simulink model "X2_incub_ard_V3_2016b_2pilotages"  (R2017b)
settings: Solver=ode45  StartTime=0.0  StopTime=35*3600  RelTol=1e-3  EnableMultiTasking=on
undefined symbols (not defined in the file or in its folder): a12fe90b, a1c04bd6127d, a1fc367dfb9e, a2a0ec7e, a4c8, a889, a952, adec, aeaa, af92, b19e, b27f, b35c, b3e0, b3e1, beff, c20252f1455d, c375904d, c5628deb, c6119d757cc9, circulargauge, continuousknob, d0c8, d78370d7, e8b45f5d51c6, eec73065, f50e, f641dc3b1927, fb31cb14, fbd800df, fec15dcb, ff27feb4, lamp, lineargauge, ninetydegreegauge, rockerswitch, semicirculargauge, serial, X2_incub_ard_V3_2016b_2pilotages
libraries: instrumentlib x4, powerlib_meascontrol x1, simulink x1, visionstatistics x1

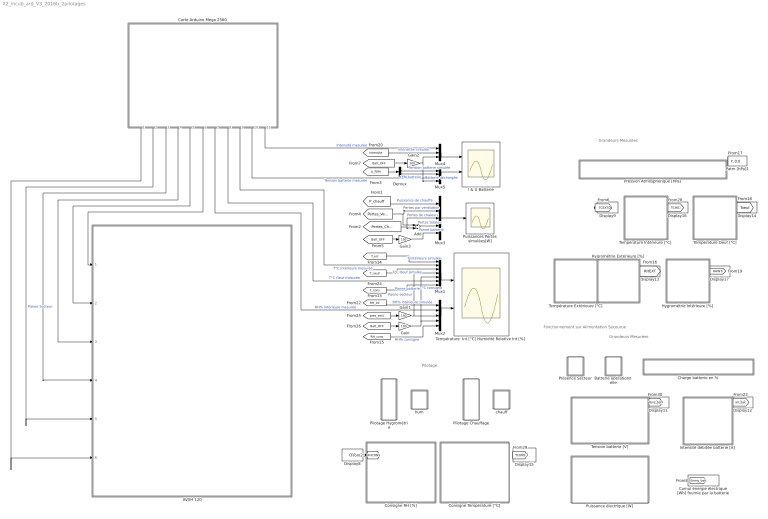
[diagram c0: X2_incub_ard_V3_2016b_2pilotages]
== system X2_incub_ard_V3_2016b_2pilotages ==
  note: Fonctionnement sur Alimentation Secourue
  note: Grandeurs Mesurées
  note: Pilotage
  note: Grandeurs Mesurées
  AVXH 120 : Subsystem
  Add : Sum
  Batterie opérationnelle : Subsystem  DialogController=hmiCreateDDGDialog  IsWebBlock=on  mask(MWDashboardBlock){webBlockId=a2a0ec7e-f50e-4eba-a952-78d570a106d8, webBlockType=lamp, ShowInLibBrowser=on, ShowInitialText=on, HMISrcModelName=X2_incub_ard_V3_2016b_2pilotages}
      mask prompts: webBlockType "WebBlock Type"; HMISrcModelName "Source Model"
  Carte Arduino Mega 2560 : Subsystem
  Charge batterie en % : Subsystem  DialogController=hmiCreateDDGDialog  IsWebBlock=on  mask(MWDashboardBlock){webBlockId=4aa34d54-a889-4dd9-8e9d-c6119d757cc9, webBlockType=lineargauge, ShowInLibBrowser=on, ShowInitialText=on, HMISrcModelName=X2_incub_ard_V3_2016b_2pilotages}
      mask prompts: webBlockId "WebBlock Id"; webBlockType "WebBlock Type"; HMISrcModelName "Source Model"
  Consigne RH [%] : Subsystem  DialogController=hmiCreateDDGDialog  IsWebBlock=on  mask(MWDashboardBlock){webBlockId=d78370d7-5ba0-404a-9b06-f641dc3b1927, webBlockType=continuousknob, ShowInLibBrowser=on, ShowInitialText=on, HMISrcModelName=X2_incub_ard_V3_2016b_2pilotages}
      mask prompts: webBlockId "WebBlock Id"; webBlockType "WebBlock Type"; HMISrcModelName "Source Model"
  Consigne Température [°C] : Subsystem  DialogController=hmiCreateDDGDialog  IsWebBlock=on  mask(MWDashboardBlock){webBlockId=fb31cb14-b3e1-42d9-b27f-609e25656f7b, webBlockType=continuousknob, ShowInLibBrowser=on, ShowInitialText=on, HMISrcModelName=X2_incub_ard_V3_2016b_2pilotages}
      mask prompts: webBlockId "WebBlock Id"; webBlockType "WebBlock Type"; HMISrcModelName "Source Model"
  Cumul énergie électrique [Wh] fournie par la batterie : Display
  Demux : Demux  Outputs=2
  Display{8..9,11..17} (9 alike) : Display
  Gain{,1..3} (4 alike) : Gain  Gain=100
  Hygrométrie Extérieure [%] : Subsystem  DialogController=hmiCreateDDGDialog  IsWebBlock=on  mask(MWDashboardBlock){webBlockId=85124ee6-0488-45a4-8674-7bc48321bb2f, webBlockType=circulargauge, ShowInLibBrowser=on, ShowInitialText=on, HMISrcModelName=X2_incub_ard_V3_2016b_2pilotages}
      mask prompts: webBlockId "WebBlock Id"; webBlockType "WebBlock Type"; HMISrcModelName "Source Model"
  Hygrométrie Intérieure [%] : Subsystem  DialogController=hmiCreateDDGDialog  IsWebBlock=on  mask(MWDashboardBlock){webBlockId=55eca8da-3471-4297-9a8a-dfdafd65951c, webBlockType=circulargauge, ShowInLibBrowser=on, ShowInitialText=on, HMISrcModelName=X2_incub_ard_V3_2016b_2pilotages}
      mask prompts: webBlockId "WebBlock Id"; webBlockType "WebBlock Type"; HMISrcModelName "Source Model"
  I & U Batterie : Scope  NumInputPorts=2
  Intensité débitée batterie [A] : Subsystem  DialogController=hmiCreateDDGDialog  IsWebBlock=on  mask(MWDashboardBlock){webBlockId=c5d743be-d443-4bfc-aabc-91b17bac25af, webBlockType=ninetydegreegauge, ShowInLibBrowser=on, ShowInitialText=on, HMISrcModelName=X2_incub_ard_V3_2016b_2pilotages}
      mask prompts: webBlockId "WebBlock Id"; webBlockType "WebBlock Type"; HMISrcModelName "Source Model"
  Mux1 : Mux  Inputs=7
  Mux2 : Mux  Inputs=5
  Mux3 : Mux  Inputs=5
  Mux4 : Mux  Inputs=3
  Mux5 : Mux
  Patm [hPa]1 : Display
  Pilotage Chauffage : Subsystem  DialogController=hmiCreateDDGDialog  IsWebBlock=on  mask(MWDashboardBlock){webBlockId=73ff47ba-1fd1-47b3-beff-c20252f1455d, webBlockType=rockerswitch, ShowInLibBrowser=on, ShowInitialText=on, HMISrcModelName=X2_incub_ard_V3_2016b_2pilotages}
      mask prompts: webBlockId "WebBlock Id"; webBlockType "WebBlock Type"; HMISrcModelName "Source Model"
  Pilotage Hygrométrie : Subsystem  DialogController=hmiCreateDDGDialog  IsWebBlock=on  mask(MWDashboardBlock){webBlockId=eec73065-76b4-4396-95f8-9ce9c4219b5b, webBlockType=rockerswitch, ShowInLibBrowser=on, ShowInitialText=on, HMISrcModelName=X2_incub_ard_V3_2016b_2pilotages}
      mask prompts: webBlockId "WebBlock Id"; webBlockType "WebBlock Type"; HMISrcModelName "Source Model"
  Pression Atmosphérique [hPa] : Subsystem  DialogController=hmiCreateDDGDialog  IsWebBlock=on  mask(MWDashboardBlock){webBlockId=ff27feb4-648a-4a8f-a4c8-0cec62a88610, webBlockType=lineargauge, ShowInLibBrowser=on, ShowInitialText=on, HMISrcModelName=X2_incub_ard_V3_2016b_2pilotages}
      mask prompts: webBlockId "WebBlock Id"; webBlockType "WebBlock Type"; HMISrcModelName "Source Model"
  Présence Secteur : Subsystem  DialogController=hmiCreateDDGDialog  IsWebBlock=on  mask(MWDashboardBlock){webBlockId=fbd800df-7ee0-4b30-9971-11a92cd70363, webBlockType=lamp, ShowInLibBrowser=on, ShowInitialText=on, HMISrcModelName=X2_incub_ard_V3_2016b_2pilotages}
      mask prompts: webBlockType "WebBlock Type"; HMISrcModelName "Source Model"
  Puissance électrique [W] : Subsystem  DialogController=hmiCreateDDGDialog  IsWebBlock=on  mask(MWDashboardBlock){webBlockId=66e2f3cb-b3e0-4f9e-b35c-a1fc367dfb9e, webBlockType=semicirculargauge, ShowInLibBrowser=on, ShowInitialText=on, HMISrcModelName=X2_incub_ard_V3_2016b_2pilotages}
      mask prompts: webBlockId "WebBlock Id"; webBlockType "WebBlock Type"; HMISrcModelName "Source Model"
  Puissances Pertes simulées[W] : Scope
  Température Extérieure [°C] : Subsystem  DialogController=hmiCreateDDGDialog  IsWebBlock=on  mask(MWDashboardBlock){webBlockId=50da628d-71fe-4d11-adec-82087158e38d, webBlockType=circulargauge, ShowInLibBrowser=on, ShowInitialText=on, HMISrcModelName=X2_incub_ard_V3_2016b_2pilotages}
      mask prompts: webBlockId "WebBlock Id"; webBlockType "WebBlock Type"; HMISrcModelName "Source Model"
  Température Intérieure [°C] : Subsystem  DialogController=hmiCreateDDGDialog  IsWebBlock=on  mask(MWDashboardBlock){webBlockId=fec15dcb-6932-4718-af92-a1c04bd6127d, webBlockType=circulargauge, ShowInLibBrowser=on, ShowInitialText=on, HMISrcModelName=X2_incub_ard_V3_2016b_2pilotages}
      mask prompts: webBlockId "WebBlock Id"; webBlockType "WebBlock Type"; HMISrcModelName "Source Model"
  Température  Int [°C] Humidité Relative Int [%] : Scope  NumInputPorts=2
  Température Oeuf [°C] : Subsystem  DialogController=hmiCreateDDGDialog  IsWebBlock=on  mask(MWDashboardBlock){webBlockId=01d8dc64-393f-4bf0-a17e-dbfae9f3e832, webBlockType=circulargauge, ShowInLibBrowser=on, ShowInitialText=on, HMISrcModelName=X2_incub_ard_V3_2016b_2pilotages}
      mask prompts: webBlockId "WebBlock Id"; webBlockType "WebBlock Type"; HMISrcModelName "Source Model"
  Tension batterie [V] : Subsystem  DialogController=hmiCreateDDGDialog  IsWebBlock=on  mask(MWDashboardBlock){webBlockId=c375904d-d0c8-4efe-9d67-62ecafe94817, webBlockType=semicirculargauge, ShowInLibBrowser=on, ShowInitialText=on, HMISrcModelName=X2_incub_ard_V3_2016b_2pilotages}
      mask prompts: webBlockId "WebBlock Id"; webBlockType "WebBlock Type"; HMISrcModelName "Source Model"
  chauff : Subsystem  DialogController=hmiCreateDDGDialog  IsWebBlock=on  mask(MWDashboardBlock){webBlockId=c5628deb-b19e-496e-84ad-10548b031044, webBlockType=lamp, ShowInLibBrowser=on, ShowInitialText=on, HMISrcModelName=X2_incub_ard_V3_2016b_2pilotages}
      mask prompts: webBlockType "WebBlock Type"; HMISrcModelName "Source Model"
  hum : Subsystem  DialogController=hmiCreateDDGDialog  IsWebBlock=on  mask(MWDashboardBlock){webBlockId=a12fe90b-90f1-46e1-aeaa-e8b45f5d51c6, webBlockType=lamp, ShowInLibBrowser=on, ShowInitialText=on, HMISrcModelName=X2_incub_ard_V3_2016b_2pilotages}
      mask prompts: webBlockType "WebBlock Type"; HMISrcModelName "Source Model"
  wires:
  [T_int] -> Mux1/1  "T intérieure simulée"
  [Intensite] -> Mux4/2  "Intensitée simulée"
  [RH_int] -> Mux2/1  "RH% intérieure simulée"
  Gain1/1 -> Mux1/4, Mux2/3  "Panne secteur"
  [pres_sect] -> Gain1/1
  [Batt_OFF] -> Gain/1
  Gain/1 -> Mux1/5, Mux2/4  "Panne batterie"
  Demux/1 -> Mux5/1  "Tension batterie simulée"
  [T_cons] -> Mux1/7  "T°C consigne"
  Carte Arduino Mega 2560/1(Patm) -> AVXH 120/6(In6)
  Mux1/1 -> Température  Int [°C] Humidité Relative Int [%]/1
  Mux2/1 -> Température  Int [°C] Humidité Relative Int [%]/2
  [P_chauff] -> Mux3/1  "Puissance de chauffe"
  [Pertes_Vent] -> Add/1, Mux3/2  "Pertes par ventilation"
  Mux3/1 -> Puissances Pertes simulées[W]/1
  [Pertes_Chaleur] -> Mux3/3, Add/2  "Pertes de chaleurs"
  Add/1 -> Mux3/4  "Pertes totales"
  [T_oeuf] -> Mux1/3  "T°C Oeuf simulée"
  Carte Arduino Mega 2560/9(T°C INT) -> Mux1/2  "T°C intérieure mesurée"
  Carte Arduino Mega 2560/7(RH% INT) -> Mux2/2  "RH% intérieure mesurée"
  Carte Arduino Mega 2560/4(RH% EXT) -> AVXH 120/3(In4)
  Carte Arduino Mega 2560/3(T°C EXT) -> AVXH 120/4(In5)
  Carte Arduino Mega 2560/2(Pres Sect) -> AVXH 120/5(Présence secteur)  "Panne Secteur"
  [RH_cons] -> Mux2/5  "RH% consigne"
  Carte Arduino Mega 2560/8(T°C OEUF) -> Mux1/6  "T°C Oeuf mesurée"
  Carte Arduino Mega 2560/5(RH Cons) -> AVXH 120/2(In3)
  Carte Arduino Mega 2560/6(T°C Cons) -> AVXH 120/1(In2)
  [RHCONS] -> Display8/1
  [TCONS] -> Display15/1
  [TCINT] -> Display16/1
  [P_atm] -> Patm [hPa]1/1
  [TCEXT] -> Display9/1
  [Toeuf] -> Display14/1
  [RHINT] -> Display17/1
  [RHEXT] -> Display13/1
  [Int_bat] -> Display12/1
  [Tens_bat] -> Display11/1
  Mux4/1 -> I & U Batterie/1
  Mux5/1 -> I & U Batterie/2
  Carte Arduino Mega 2560/11(I) -> Mux4/1  "Intensité mesurée"
  Carte Arduino Mega 2560/10(U) -> Mux5/3  "Tension batterie mesurée"
  [U_FEM] -> Demux/1
  Demux/2 -> Mux5/2  "FEM batterie"
  [Batt_OFF] -> Gain2/1
  Gain2/1 -> Mux5/4, Mux4/3  "Batterie déchargée"
  [Batt_OFF] -> Gain3/1
  Gain3/1 -> Mux3/5  "Panne batterie"
  [Energ_batt] -> Cumul énergie électrique [Wh] fournie par la batterie/1

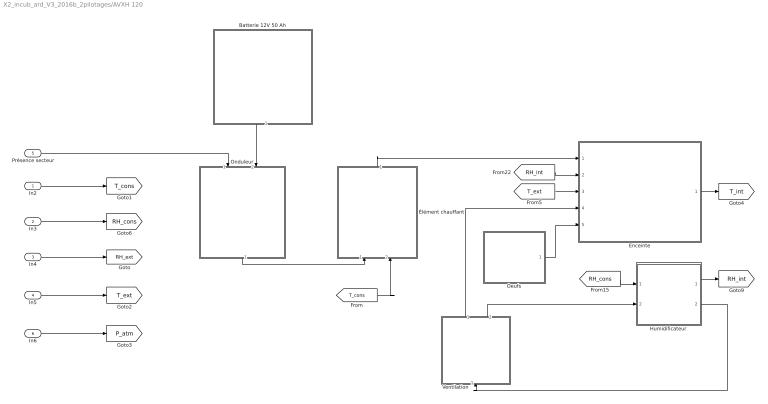
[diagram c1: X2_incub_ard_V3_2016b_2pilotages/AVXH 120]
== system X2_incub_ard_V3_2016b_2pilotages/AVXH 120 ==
  In2 : Inport
  In3 : Inport  Port=2
  In4 : Inport  Port=3
  In5 : Inport  Port=4
  Présence secteur : Inport  Port=5
  In6 : Inport  Port=6
  Batterie 12V 50 Ah : Subsystem  mask{V0=12.8, Icc=400, C0=50, C1=20, V1=12.1}
      mask prompts: V0 "Tension nominale [V]"; Icc "Intensité de Court Circuit [A]"; C0 "Capacité Totale [Ah]"; C1 "Charge C1 à V1 [Ah]"; V1 "Tension V1 à C1 [V]"
  Enceinte : Subsystem  mask{V=88.3, R_iso=0.38}
      mask prompts: V "Volume interne [litre]"; R_iso "Résistance thermique isolant [m².K/W]"
  Humidificateur : Subsystem
  Oeufs : Subsystem  mask{Nbre=1}
      mask prompts: Nbre "Nombre d'oeufs"
  Onduleur : Subsystem
  Ventilation : Subsystem  mask{Qair=0.63, Qpanne=0.02}
  Élément chauffant : Subsystem
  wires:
  [RH_int] -> Enceinte/2(In2)
  Enceinte/1(T°C in) -> [T_int]
  Présence secteur/1 -> Onduleur/1(In1)
  In6/1 -> [P_atm]
  In5/1 -> [T_ext]
  [T_ext] -> Enceinte/3(T°C ext)
  In4/1 -> [RH_ext]
  In3/1 -> [RH_cons]
  Oeufs/1(Out1) -> Enceinte/5(M.Cp_Oeuf)
  Élément chauffant/1(Out2) -> Enceinte/1(P_chauff)
  Ventilation/1(Out1) -> Enceinte/4(Pertes ventilation)
  [RH_cons] -> Humidificateur/1(In1)
  Ventilation/2(Out2) -> Humidificateur/2(In2)
  Humidificateur/2(Out2) -> Ventilation/1(In1)
  In2/1 -> [T_cons]
  Batterie 12V 50 Ah/1(Out3) -> Onduleur/2(In2)
  Onduleur/1(Out1) -> Élément chauffant/1(In1)
  [T_cons] -> Élément chauffant/2(In2)
  Humidificateur/1(Out1) -> [RH_int]

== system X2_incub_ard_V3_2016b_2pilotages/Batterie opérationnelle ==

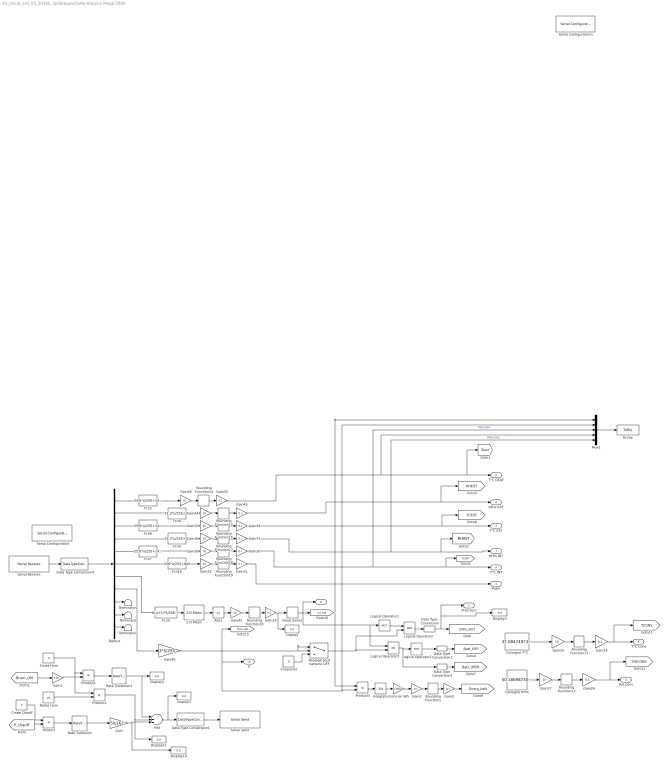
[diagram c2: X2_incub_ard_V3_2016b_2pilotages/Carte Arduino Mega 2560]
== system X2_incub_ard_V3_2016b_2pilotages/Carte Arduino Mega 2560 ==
  2-D Mean : visionstatistics/2-D Mean  run=on  reset_popup=None  directionMode=Entire input  dimension=1  treatSBRowAsCol=on  roiEnable=off  roiType=Rectangles  roiPortion=Entire ROI  roiOutput=Individual statistics for each ROI  roiFlag=off  outputDataTypeStr=Inherit: Same as accumulator  outputLastDataTypeStr=Inherit: Same as accumulator  outputMin=[]  outputMax=[]  accumMode=Binary point scaling  accumWordLength=32  accumFracLength=0  accumDataTypeStr=fixdt([],32,0)  accumLastDataTypeStr=fixdt([],32,0)  roundingMode=Floor  overflowMode=off
  Abs1 : Abs
  Add : Sum  Inputs=+++
  Cmde Chauff : Constant  Value=0  SampleTime=1
  Cmde Hum : Constant  Value=0  SampleTime=1
  Consigne RH% : Constant  Value=50.1869873046875
  Consigne T°C : Constant  Value=37.084749730428
  Constant2 : Constant  Value=0
  Conv en Wh : Gain  Gain=1/3600
  Data Type Conversion{,1,3..4} (4 alike) : DataTypeConversion  OutDataTypeStr=double
  Data Type Conversion5 : DataTypeConversion  OutDataTypeStr=uint8
  Dead Zone1 : DeadZone  LowerValue=0  UpperValue=0.6
  Demux : Demux  Outputs=11
  Display{,1..3,10..11} (6 alike) : Display
  Fcn10 : Fcn  Expr=256*u/255+845
  Fcn2 : Fcn  Expr=25.6*u/255+14.4
  Fcn5 : Fcn  Expr=((u+2)*5/256-2.5)/0.0833
  Fcn6 : Fcn  Expr=25.6*u/255+14.4
  Fcn7 : Fcn  Expr=25.6*u/255+14.4
  Fcn8 : Fcn  Expr=51.2*u/255+35
  Fcn9 : Fcn  Expr=51.2*u/255+35
  Gain : Gain  Gain=50/162
  Gain1 : Gain  Gain=120
  Gain{2,24,26,29..31,34..35,37,45} (10 alike) : Gain  Gain=0.1
  Gain{3,25,27,32..33,36,38,42,44,46} (10 alike) : Gain  Gain=10
  Gain40 : Gain  Gain=3*5/255
  Integrator : Integrator
  Logical Operator1 : Logic  Operator=NOT  AllPortsSameDT=off  OutDataTypeStr=boolean
  Logical Operator2 : Logic  AllPortsSameDT=off  OutDataTypeStr=boolean
  Logical Operator3 : Logic  Operator=OR  AllPortsSameDT=off  OutDataTypeStr=boolean
  Logical Operator5 : Logic  Operator=NOT  AllPortsSameDT=off  OutDataTypeStr=boolean
  Mux1 : Mux  Inputs=5
  Product{,1..3} (4 alike) : Product
  Rate Transition : RateTransition  OutPortSampleTime=1
  Rate Transition1 : RateTransition  OutPortSampleTime=1
  Relais Hum : Constant  Value=60  SampleTime=1
  Rounding Function{1,11..12,14..20} (10 alike) : Rounding  Operator=round
  Réglage seuil batterie OFF : Switch  Criteria=u2 > Threshold  Threshold=11.5
  Serial Configuration : instrumentlib/Serial Configuration  Priority=-200000  ComPortMenu=<Please select a port...>  ComPort=<Please select a port...>  BaudRate=9600  DataBits=8  Parity=none  StopBits=1  FlowControl=none  Timeout=10  ByteOrder=LittleEndian
  Serial Configuration1 : instrumentlib/Serial Configuration  Priority=-200000  ComPortMenu=COM18  ComPort=COM18  ObjConstructor=serial('COM18');  BaudRate=9600  DataBits=8  Parity=none  StopBits=1  FlowControl=none  Timeout=10  ByteOrder=LittleEndian
  Serial Receive : instrumentlib/Serial Receive  ComPortMenu=COM18  ComPort=COM18  ObjConstructor=serial('COM18');  Terminator=<none>  DataSize="[1  11]"  DataType=uint8  EnableBlockingMode=on  ActionDataUnavailable=Output last received value  CustomValue=0  SampleTime=1
  Serial Send : instrumentlib/Serial Send  ComPortMenu=COM18  ComPort=COM18  ObjConstructor=serial('COM18');  Terminator=<none>  EnableBlockingMode=on
  Terminator : Terminator
  Terminator1 : Terminator
  Terminator2 : Terminator
  To File : ToFile  Filename=mesures.mat  SaveFormat=Timeseries
  Patm : Outport
  Pres Sect : Outport  Port=2
  T°C EXT : Outport  Port=3
  RH% EXT : Outport  Port=4
  RH Cons : Outport  Port=5
  T°C Cons : Outport  Port=6
  RH% INT : Outport  Port=7
  T°C OEUF : Outport  Port=8
  T°C INT : Outport  Port=9
  U : Outport  Port=10
  I : Outport  Port=11
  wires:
  Rounding Function11/1 -> Gain24/1
  Gain25/1 -> Rounding Function11/1
  Consigne T°C/1 -> Gain25/1
  Gain24/1 -> [TCONS], T°C Cons/1
  Rounding Function12/1 -> Gain26/1
  Gain27/1 -> Rounding Function12/1
  Gain26/1 -> [RHCONS], RH Cons/1
  Consigne RH%/1 -> Gain27/1
  Mux1/1 -> To File/1
  Gain35/1 -> [Toeuf], T°C OEUF/1, Mux1/4
  Gain45/1 -> [RHEXT], RH% EXT/1
  Gain31/1 -> Patm/1
  Fcn5/1 -> 2-D Mean/1
  Demux/7 -> Fcn5/1
  Gain37/1 -> Mux1/5, RH% INT/1, [RHINT]  "Mesurée"
  Gain34/1 -> T°C EXT/1, [TCEXT]
  Gain40/1 -> [Tens_bat], Réglage seuil batterie OFF/1, Réglage seuil batterie OFF/2, Product3/2, Mux1/2, U/1
  Demux/2 -> Fcn8/1
  Demux/3 -> Fcn6/1
  Demux/4 -> Fcn9/1
  Demux/5 -> Fcn7/1
  Demux/1 -> Fcn2/1
  Fcn2/1 -> Gain46/1
  Fcn6/1 -> Gain33/1
  Fcn7/1 -> Gain38/1
  Fcn8/1 -> Gain44/1
  Fcn9/1 -> Gain36/1
  Fcn10/1 -> Gain32/1
  Rounding Function14/1 -> Gain35/1
  Gain46/1 -> Rounding Function14/1
  Rounding Function15/1 -> Gain45/1
  Gain44/1 -> Rounding Function15/1
  Rounding Function16/1 -> Gain34/1
  Gain33/1 -> Rounding Function16/1
  Rounding Function17/1 -> Gain37/1
  Gain36/1 -> Rounding Function17/1
  Rounding Function18/1 -> Gain30/1
  Gain38/1 -> Rounding Function18/1
  Rounding Function19/1 -> Gain31/1
  Gain32/1 -> Rounding Function19/1
  Serial Receive/1 -> Data Type Conversion4/1
  Data Type Conversion4/1 -> Demux/1
  Rounding Function20/1 -> Gain29/1
  Gain42/1 -> Rounding Function20/1
  Abs1/1 -> Gain42/1
  Demux/6 -> Fcn10/1
  Gain30/1 -> Mux1/3, T°C INT/1, [TCINT]  "Mesurée"
  2-D Mean/1 -> Abs1/1
  Gain/1 -> Display10/1, Add/3
  Demux/10 -> Terminator/1
  Demux/11 -> Terminator1/1
  Demux/9 -> Terminator2/1
  Data Type Conversion5/1 -> Serial Send/1
  Rate Transition/1 -> Gain/1
  Constant2/1 -> Réglage seuil batterie OFF/3
  Demux/8 -> Gain40/1
  Gain29/1 -> Display/1, Dead Zone1/1
  Réglage seuil batterie OFF/1 -> Logical Operator3/2, Logical Operator2/2
  Data Type Conversion/1 -> Pres Sect/1, Display3/1, [pres_sect]
  Dead Zone1/1 -> Mux1/1, Product3/1, Logical Operator3/1, Logical Operator1/1, I/1, [Int_bat]
  Cmde Chauff/1 -> Product/1
  Product/1 -> Rate Transition/1
  Logical Operator2/1 -> Data Type Conversion/1
  Logical Operator3/1 -> Data Type Conversion3/1, Logical Operator5/1
  Logical Operator5/1 -> Data Type Conversion1/1
  Logical Operator1/1 -> Logical Operator2/1
  Data Type Conversion1/1 -> [Batt_OFF]
  Data Type Conversion3/1 -> [Batt_OPER]
  [P_chauff] -> Product/2
  Add/1 -> Display1/1, Data Type Conversion5/1
  Cmde Hum/1 -> Product2/1, Product1/1
  [Brum_ON] -> Gain1/1
  Gain1/1 -> Product1/2
  Product1/1 -> Rate Transition1/1
  Rate Transition1/1 -> Display2/1, Add/1
  Relais Hum/1 -> Product2/2
  Product2/1 -> Display11/1, Add/2
  Product3/1 -> Integrator/1
  Integrator/1 -> Conv en Wh/1
  Conv en Wh/1 -> Gain3/1
  Rounding Function1/1 -> Gain2/1
  Gain3/1 -> Rounding Function1/1
  Gain2/1 -> [Energ_batt]

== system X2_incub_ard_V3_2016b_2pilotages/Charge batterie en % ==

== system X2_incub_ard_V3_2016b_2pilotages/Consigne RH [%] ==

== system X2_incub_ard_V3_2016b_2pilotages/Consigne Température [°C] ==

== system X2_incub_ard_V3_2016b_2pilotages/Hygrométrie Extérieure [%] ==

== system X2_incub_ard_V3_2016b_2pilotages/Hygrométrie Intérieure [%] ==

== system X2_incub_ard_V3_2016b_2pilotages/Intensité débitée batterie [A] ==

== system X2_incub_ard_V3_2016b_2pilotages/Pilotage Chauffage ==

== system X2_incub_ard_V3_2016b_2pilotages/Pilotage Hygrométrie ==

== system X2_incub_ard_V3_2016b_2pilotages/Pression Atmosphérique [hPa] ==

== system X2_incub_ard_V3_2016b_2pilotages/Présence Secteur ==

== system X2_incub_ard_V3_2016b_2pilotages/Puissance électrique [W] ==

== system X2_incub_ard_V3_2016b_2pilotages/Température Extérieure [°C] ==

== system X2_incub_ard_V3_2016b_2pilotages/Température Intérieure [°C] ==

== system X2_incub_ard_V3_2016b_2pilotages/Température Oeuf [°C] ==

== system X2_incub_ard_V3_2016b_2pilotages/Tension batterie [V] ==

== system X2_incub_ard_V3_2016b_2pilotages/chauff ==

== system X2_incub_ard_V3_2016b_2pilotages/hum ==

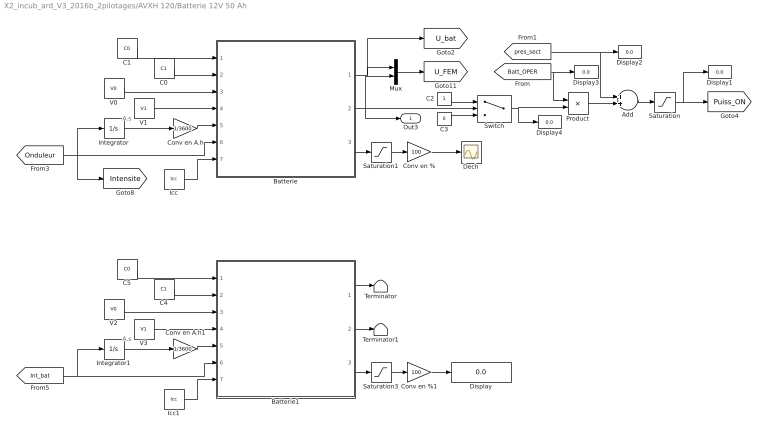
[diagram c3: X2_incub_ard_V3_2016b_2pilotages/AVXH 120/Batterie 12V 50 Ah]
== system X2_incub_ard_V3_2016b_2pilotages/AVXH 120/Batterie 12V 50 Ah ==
  note: A.s
  note: A.s
  Add : Sum
  Batterie : MATLAB Function  TreatAsAtomicUnit=on
  Batterie1 : MATLAB Function  TreatAsAtomicUnit=on
  C0 : Constant  Value=C1
  C1 : Constant  Value=C0
  C2 : Constant
  C3 : Constant  Value=0
  C4 : Constant  Value=C1
  C5 : Constant  Value=C0
  Conv en % : Gain  Gain=100
  Conv en %1 : Gain  Gain=100
  Conv en A.h : Gain  Gain=1/3600
  Conv en A.h1 : Gain  Gain=1/3600
  Dech : Scope
  Display{,1..4} (5 alike) : Display
  Icc : Constant  Value=Icc
  Icc1 : Constant  Value=Icc
  Integrator : Integrator
  Integrator1 : Integrator
  Mux : Mux  Inputs=2
  Product : Product
  Saturation : Saturate  UpperLimit=1  LowerLimit=0
  Saturation1 : Saturate  UpperLimit=1000  LowerLimit=0
  Saturation3 : Saturate  UpperLimit=1000  LowerLimit=0
  Switch : Switch  Criteria=u2 > Threshold  Threshold=11
  Terminator : Terminator
  Terminator1 : Terminator
  V0 : Constant  Value=V0
  V1 : Constant  Value=V1
  V2 : Constant  Value=V0
  V3 : Constant  Value=V1
  Out3 : Outport
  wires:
  Batterie/3(x) -> Saturation1/1
  Conv en %/1 -> Dech/1
  Batterie/1(U) -> [U_bat], Mux/1
  C0/1 -> Batterie/2(C1)
  C1/1 -> Batterie/1(C0)
  V0/1 -> Batterie/3(V0)
  V1/1 -> Batterie/4(V1)
  Icc/1 -> Batterie/7(Icc)
  Integrator/1 -> Conv en A.h/1
  Conv en A.h/1 -> Batterie/5(C)
  Mux/1 -> [U_FEM]
  C2/1 -> Switch/1
  C3/1 -> Switch/3
  Saturation1/1 -> Conv en %/1
  Switch/1 -> Display4/1, Product/2
  [Onduleur] -> [Intensite], Integrator/1, Batterie/6(I)
  Product/1 -> Add/2
  [Batt_OPER] -> Display3/1, Product/1
  Add/1 -> Saturation/1
  [pres_sect] -> Display2/1, Add/1
  Batterie/2(E) -> Mux/2, Out3/1, Switch/2
  Batterie1/3(x) -> Saturation3/1
  Conv en %1/1 -> Display/1
  C4/1 -> Batterie1/2(C1)
  C5/1 -> Batterie1/1(C0)
  V2/1 -> Batterie1/3(V0)
  V3/1 -> Batterie1/4(V1)
  Icc1/1 -> Batterie1/7(Icc)
  Integrator1/1 -> Conv en A.h1/1
  Conv en A.h1/1 -> Batterie1/5(C)
  Saturation3/1 -> Conv en %1/1
  [Int_bat] -> Batterie1/6(I), Integrator1/1
  Batterie1/1(U) -> Terminator/1
  Batterie1/2(E) -> Terminator1/1
  Saturation/1 -> Display1/1, [Puiss_ON]

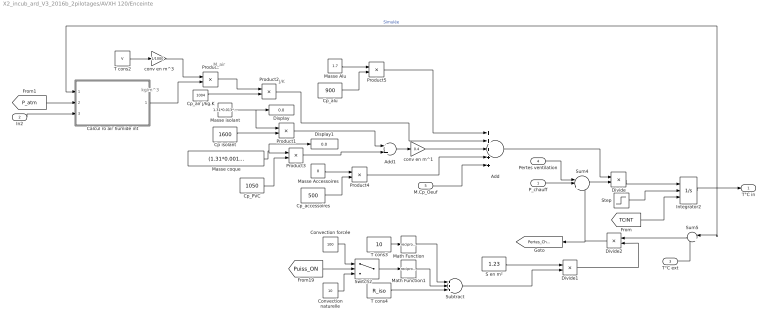
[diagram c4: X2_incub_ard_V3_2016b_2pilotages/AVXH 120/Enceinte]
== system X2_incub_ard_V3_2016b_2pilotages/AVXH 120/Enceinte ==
  note: J/K
  note: kg/m^3
  note: M_air
  P_chauff : Inport
  In2 : Inport  Port=2
  T°C ext : Inport  Port=3
  Pertes ventilation : Inport  Port=4
  M.Cp_Oeuf : Inport  Port=5
  Add : Sum  Inputs=+++++
  Add1 : Sum
  Calcul ro air humide int : MATLAB Function  TreatAsAtomicUnit=on
  Convection forcée : Constant  Value=100
  Convection naturelle : Constant  Value=10
  Cp isolant : Constant  Value=1600
  Cp_PVC : Constant  Value=1050
  Cp_accessoires : Constant  Value=500
  Cp_air j/kg.K : Constant  Value=1004
  Cp_alu : Constant  Value=900
  Display : Display
  Display1 : Display
  Divide : Product  Inputs=/*
  Divide1 : Product  Inputs=*/
  Divide2 : Product  Inputs=**
  Integrator2 : Integrator  ExternalReset=rising  InitialConditionSource=external  InitialCondition=20
  Masse Accessoires : Constant  Value=8
  Masse Alu : Constant  Value=1.7
  Masse coque : Constant  Value=(1.31*0.001+1.23*0.001)*1380
  Masse isolant : Constant  Value=1.31*0.013*40
  Math Function : Math  Operator=reciprocal
  Math Function1 : Math  Operator=reciprocal
  Product{,1..5} (6 alike) : Product
  S en m² : Constant  Value=1.23
  Step : Step  SampleTime=0
  Subtract : Sum  Inputs=+++
  Sum4 : Sum  Inputs=-|+|-
  Sum5 : Sum  Inputs=|+-
  Switch2 : Switch  Criteria=u2 > Threshold
  T cons2 : Constant  Value=V
  T cons3 : Constant  Value=10
  T cons4 : Constant  Value=R_iso
  conv en m^1 : Gain  Gain=0.4
  conv en m^3 : Gain  Gain=1/1000
  T°C in : Outport
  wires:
  P_chauff/1 -> Sum4/2
  Sum4/1 -> Divide/2
  Sum5/1 -> Divide2/1
  Divide2/1 -> Sum4/3, [Pertes_Chaleur]
  Divide/1 -> Integrator2/1
  T°C ext/1 -> Sum5/2
  T cons2/1 -> conv en m^3/1
  Calcul ro air humide int/1(RO) -> Product/2
  Product/1 -> Product2/1
  Masse isolant/1 -> Display/1, Product1/1
  Cp_air j/kg.K/1 -> Product2/2
  Cp isolant/1 -> Product1/2
  Product1/1 -> Add1/1
  Product2/1 -> Add/2
  [P_atm] -> Calcul ro air humide int/2(P)
  Add/1 -> Divide/1
  S en m²/1 -> Divide1/1
  T cons4/1 -> Subtract/3
  Divide1/1 -> Divide2/2
  In2/1 -> Calcul ro air humide int/3(RH)
  Pertes ventilation/1 -> Sum4/1
  conv en m^3/1 -> Product/1
  T cons3/1 -> Math Function/1
  Switch2/1 -> Math Function1/1
  Math Function1/1 -> Subtract/2
  Math Function/1 -> Subtract/1
  Subtract/1 -> Divide1/2
  Cp_PVC/1 -> Product3/2
  Product3/1 -> Add1/2
  Masse Accessoires/1 -> Product4/1
  Cp_accessoires/1 -> Product4/2
  Product4/1 -> Add/4
  Masse Alu/1 -> Product5/1
  Cp_alu/1 -> Product5/2
  Product5/1 -> Add/1
  M.Cp_Oeuf/1 -> Add/5
  [TCINT] -> Integrator2/3
  Masse coque/1 -> Display1/1, Product3/1
  Integrator2/1 -> Sum5/1, Calcul ro air humide int/1(T), T°C in/1  "Simulée"
  Add1/1 -> conv en m^1/1
  conv en m^1/1 -> Add/3
  Convection forcée/1 -> Switch2/1
  Convection naturelle/1 -> Switch2/3
  [Puiss_ON] -> Switch2/2
  Step/1 -> Integrator2/2

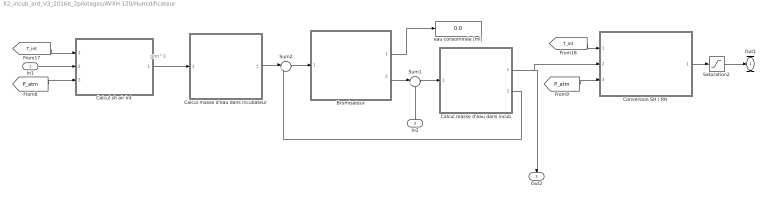
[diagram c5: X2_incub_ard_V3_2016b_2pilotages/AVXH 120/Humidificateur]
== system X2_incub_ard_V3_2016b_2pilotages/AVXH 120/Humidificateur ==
  note: g/m^3
  In1 : Inport
  In2 : Inport  Port=2
  Brumisateur : Subsystem
  Calcul masse d'eau dans incub : Subsystem
  Calcul masse d'eau dans incubateur : Subsystem
  Calcul sh air int : MATLAB Function  TreatAsAtomicUnit=on
  Conversion SH / RH : MATLAB Function  TreatAsAtomicUnit=on
  Saturation2 : Saturate  UpperLimit=100  LowerLimit=0
  Sum1 : Sum  Inputs=|++
  Sum2 : Sum  Inputs=|+-
  eau consommée [ml] : Display
  Out1 : Outport
  Out2 : Outport  Port=2
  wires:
  Sum2/1 -> Brumisateur/1(In1)
  [P_atm] -> Calcul sh air int/3(pl)
  Conversion SH / RH/1(rh) -> Saturation2/1
  Brumisateur/2(Out2) -> Sum1/1
  In1/1 -> Calcul sh air int/2(rh)
  Calcul sh air int/1(sh) -> Calcul masse d'eau dans incubateur/1(In1)
  Calcul masse d'eau dans incub/1(Out1) -> Out2/1, Conversion SH / RH/2(sh)
  Sum1/1 -> Calcul masse d'eau dans incub/1(In1)
  [T_int] -> Calcul sh air int/1(T)
  Calcul masse d'eau dans incubateur/1(Out1) -> Sum2/1
  In2/1 -> Sum1/2
  [T_int] -> Conversion SH / RH/1(T)
  [P_atm] -> Conversion SH / RH/3(pl)
  Brumisateur/1(Q eau consommée (ml)) -> eau consommée [ml]/1
  Calcul masse d'eau dans incub/2(Out2) -> Sum2/2
  Saturation2/1 -> Out1/1

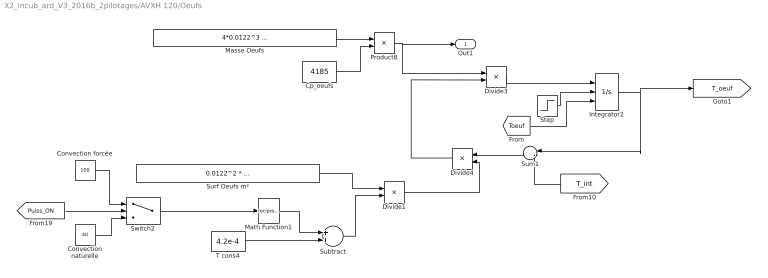
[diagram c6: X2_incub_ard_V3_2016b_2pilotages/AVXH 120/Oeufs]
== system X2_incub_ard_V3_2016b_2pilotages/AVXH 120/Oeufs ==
  Convection forcée : Constant  Value=100
  Convection naturelle : Constant  Value=40
  Cp_oeufs : Constant  Value=4185
  Divide1 : Product  Inputs=*/
  Divide3 : Product  Inputs=/*
  Divide4 : Product  Inputs=**
  Integrator2 : Integrator  ExternalReset=rising  InitialConditionSource=external  InitialCondition=20
  Masse Oeufs : Constant  Value=4*0.0122^3 * (3.14 * (3 - 1.4142) - 1) * 1000 * Nbre / 3
  Math Function1 : Math  Operator=reciprocal
  Product8 : Product
  Step : Step  SampleTime=0
  Subtract : Sum
  Sum1 : Sum  Inputs=|-+
  Surf Oeufs m² : Constant  Value=0.0122^2 * (3.14 * (3 - 1.4142) - 1) * Nbre
  Switch2 : Switch  Criteria=u2 > Threshold  Threshold=0.5
  T cons4 : Constant  Value=4.2e-4
  Out1 : Outport
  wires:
  Cp_oeufs/1 -> Product8/2
  Masse Oeufs/1 -> Product8/1
  Product8/1 -> Out1/1, Divide3/1
  Divide4/1 -> Divide3/2
  [Toeuf] -> Integrator2/3
  Integrator2/1 -> [T_oeuf], Sum1/1
  Sum1/1 -> Divide4/1
  T cons4/1 -> Subtract/2
  Divide1/1 -> Divide4/2
  Math Function1/1 -> Subtract/1
  Subtract/1 -> Divide1/2
  [T_int] -> Sum1/2
  Divide3/1 -> Integrator2/1
  Surf Oeufs m²/1 -> Divide1/1
  Convection forcée/1 -> Switch2/1
  Convection naturelle/1 -> Switch2/3
  [Puiss_ON] -> Switch2/2
  Switch2/1 -> Math Function1/1
  Step/1 -> Integrator2/2

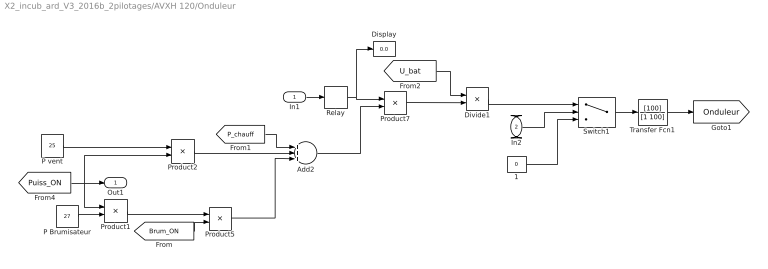
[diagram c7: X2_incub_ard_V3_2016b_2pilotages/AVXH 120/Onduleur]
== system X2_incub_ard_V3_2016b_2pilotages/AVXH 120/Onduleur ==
  In1 : Inport
  In2 : Inport  Port=2
  1 : Constant  Value=0
  Add2 : Sum  Inputs=+++
  Display : Display
  Divide1 : Product  Inputs=/*
  P Brumisateur : Constant  Value=27
  P vent : Constant  Value=25
  Product{1..2,5,7} (4 alike) : Product
  Relay : Relay  OnSwitchValue=1  OffSwitchValue=0  OnOutputValue=0  OffOutputValue=1
  Switch1 : Switch  Threshold=11
  Transfer Fcn1 : TransferFcn  Numerator=[100]  Denominator=[1 100]
  Out1 : Outport
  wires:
  Relay/1 -> Display/1, Product7/1
  Add2/1 -> Product7/2
  Product2/1 -> Add2/2
  [Brum_ON] -> Product5/2
  P Brumisateur/1 -> Product1/2
  Product5/1 -> Add2/3
  In1/1 -> Relay/1
  [P_chauff] -> Add2/1
  Divide1/1 -> Switch1/1
  1/1 -> Switch1/3
  Product7/1 -> Divide1/2
  [U_bat] -> Divide1/1
  Switch1/1 -> Transfer Fcn1/1
  In2/1 -> Switch1/2
  [Puiss_ON] -> Product1/1, Out1/1, Product2/2
  Product1/1 -> Product5/1
  P vent/1 -> Product2/1
  Transfer Fcn1/1 -> [Onduleur]

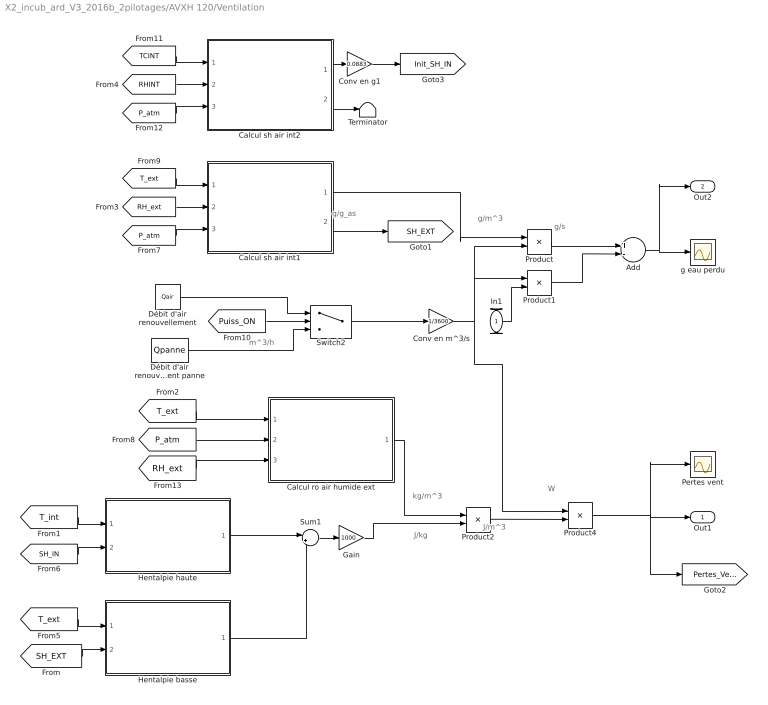
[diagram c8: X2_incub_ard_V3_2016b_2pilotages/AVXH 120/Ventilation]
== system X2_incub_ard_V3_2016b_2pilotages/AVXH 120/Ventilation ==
  note: g/g_as
  note: g/s
  note: W
  note: J/m^3
  note: kg/m^3
  note: J/kg
  note: g/m^3
  note: m^3/h
  In1 : Inport
  Add : Sum  Inputs=+-
  Calcul ro air humide ext : MATLAB Function  TreatAsAtomicUnit=on
  Calcul sh air int1 : MATLAB Function  TreatAsAtomicUnit=on
  Calcul sh air int2 : MATLAB Function  TreatAsAtomicUnit=on
  Conv en g1 : Gain  Gain=0.0883
  Conv en m^3/s : Gain  Gain=1/3600
  Débit d'air renouvellement : Constant  Value=Qair
  Débit d'air renouvellement panne : Constant  Value=Qpanne
  Gain : Gain  Gain=1000
  Hentalpie basse : MATLAB Function  TreatAsAtomicUnit=on
  Hentalpie haute : MATLAB Function  TreatAsAtomicUnit=on
  Pertes vent : Scope
  Product{,1..2,4} (4 alike) : Product
  Sum1 : Sum  Inputs=|+-
  Switch2 : Switch  Criteria=u2 > Threshold
  Terminator : Terminator
  g eau perdu : Scope
  Out1 : Outport
  Out2 : Outport  Port=2
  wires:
  Add/1 -> Out2/1, g eau perdu/1
  Switch2/1 -> Conv en m^3/s/1
  Conv en m^3/s/1 -> Product1/1, Product/2, Product4/1
  Product/1 -> Add/1
  Product1/1 -> Add/2
  Calcul ro air humide ext/1(RO) -> Product2/1
  Product2/1 -> Product4/2
  Débit d'air renouvellement/1 -> Switch2/1
  Débit d'air renouvellement panne/1 -> Switch2/3
  [Puiss_ON] -> Switch2/2
  [T_ext] -> Calcul ro air humide ext/1(T)
  [T_ext] -> Calcul sh air int1/1(T)
  [P_atm] -> Calcul sh air int1/3(pl)
  [P_atm] -> Calcul ro air humide ext/2(P)
  [RH_ext] -> Calcul sh air int1/2(rh)
  [RH_ext] -> Calcul ro air humide ext/3(RH)
  Product4/1 -> [Pertes_Vent], Out1/1, Pertes vent/1
  In1/1 -> Product1/2
  Gain/1 -> Product2/2
  [T_int] -> Hentalpie haute/1(T)
  [T_ext] -> Hentalpie basse/1(T)
  [SH_EXT] -> Hentalpie basse/2(SH)
  [SH_IN] -> Hentalpie haute/2(SH)
  Hentalpie haute/1(H1) -> Sum1/1
  Hentalpie basse/1(H1) -> Sum1/2
  Sum1/1 -> Gain/1
  Calcul sh air int1/2(sh2) -> [SH_EXT]
  [RHINT] -> Calcul sh air int2/2(rh)
  [TCINT] -> Calcul sh air int2/1(T)
  [P_atm] -> Calcul sh air int2/3(pl)
  Calcul sh air int2/1(sh) -> Conv en g1/1
  Conv en g1/1 -> [Init_SH_IN]
  Calcul sh air int1/1(sh) -> Product/1
  Calcul sh air int2/2(sh2) -> Terminator/1

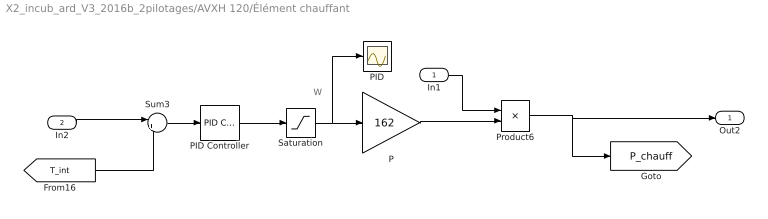
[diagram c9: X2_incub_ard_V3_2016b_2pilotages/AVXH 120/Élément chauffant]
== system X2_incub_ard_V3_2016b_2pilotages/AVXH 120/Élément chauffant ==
  note: W
  In1 : Inport
  In2 : Inport  Port=2
  P : Gain  Gain=162
  PID : Scope
  PID Controller : simulink/Continuous/PID Controller  Controller=PID  TimeDomain=Continuous-time  SampleTime=-1  IntegratorMethod=Forward Euler  FilterMethod=Forward Euler  Form=Parallel  UseFilter=on  ControllerParametersSource=internal  P=0.0897573355031779  I=3.41688472569394e-05  D=-22.2891464593491  N=0.00402695256486726  InitialConditionSource=internal  InitialConditionForIntegrator=0  InitialConditionForFilter=0  ExternalReset=none  LimitOutput=off  UpperSaturationLimit=inf  LowerSaturationLimit=-inf  LinearizeAsGain=on  AntiWindupMode=none  Kb=1  TrackingMode=off  Kt=1  PParamMin=[]  PParamMax=[]  IParamMin=[]  IParamMax=[]  DParamMin=[]  DParamMax=[]  NParamMin=[]  NParamMax=[]  KbParamMin=[]  KbParamMax=[]  KtParamMin=[]  KtParamMax=[]  POutMin=[]  POutMax=[]  IOutMin=[]  IOutMax=[]  DOutMin=[]  DOutMax=[]  NOutMin=[]  NOutMax=[]  KbOutMin=[]  KbOutMax=[]  KtOutMin=[]  KtOutMax=[]  IntegratorOutMin=[]  IntegratorOutMax=[]  FilterOutMin=[]  FilterOutMax=[]  SumOutMin=[]  SumOutMax=[]  SumI1OutMin=[]  SumI1OutMax=[]  SumI2OutMin=[]  SumI2OutMax=[]  SumI3OutMin=[]  SumI3OutMax=[]  SumDOutMin=[]  SumDOutMax=[]  SaturationOutMin=[]  SaturationOutMax=[]  IntegratorContinuousStateAttributes=''  IntegratorStateMustResolveToSignalObject=off  IntegratorRTWStateStorageClass=Auto  FilterContinuousStateAttributes=''  FilterStateMustResolveToSignalObject=off  FilterRTWStateStorageClass=Auto  DifferentiatorICPrevScaledInput=0  DifferentiatorOutMin=[]  DifferentiatorOutMax=[]  InitialConditionSetting=State (most efficient)  FilterDiffOutCoefMin=[]  FilterDiffOutCoefMax=[]  SumDenOutMin=[]  SumDenOutMax=[]  SumNumOutMin=[]  SumNumOutMax=[]  ReciprocalOutMin=[]  ReciprocalOutMax=[]  DivideOutMin=[]  DivideOutMax=[]  TunerSelectOption=Transfer Function Based (PID Tuner App)
  Product6 : Product
  Saturation : Saturate  UpperLimit=1  LowerLimit=0
  Sum3 : Sum  Inputs=|+-
  Out2 : Outport
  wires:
  In2/1 -> Sum3/1
  PID Controller/1 -> Saturation/1
  Sum3/1 -> PID Controller/1
  Saturation/1 -> PID/1, P/1
  Product6/1 -> [P_chauff], Out2/1
  [T_int] -> Sum3/2
  In1/1 -> Product6/1
  P/1 -> Product6/2

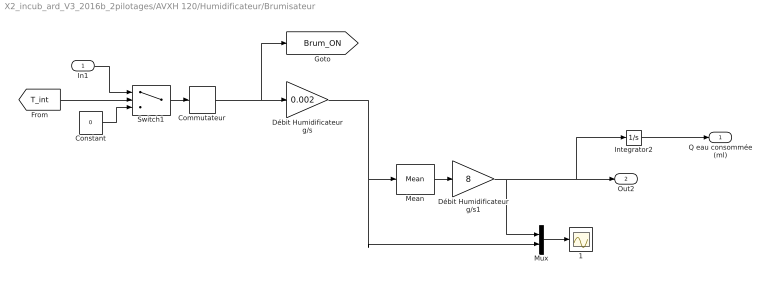
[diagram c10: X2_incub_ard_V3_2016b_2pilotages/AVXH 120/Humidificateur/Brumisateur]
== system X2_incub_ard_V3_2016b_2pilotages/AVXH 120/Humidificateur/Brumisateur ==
  In1 : Inport
  1 : Scope
  Commutateur : Relay  OnSwitchValue=0.11  OffSwitchValue=-0.02
  Constant : Constant  Value=0
  Débit Humidificateur g/s : Gain  Gain=0.002
  Débit Humidificateur g/s1 : Gain  Gain=8
  Integrator2 : Integrator
  Mean : powerlib_meascontrol/Measurements/Mean  Freq=0.061  Vinit=0  Ts=0
  Mux : Mux  Inputs=2
  Switch1 : Switch  Criteria=u2 > Threshold  Threshold=25
  Q eau consommée (ml) : Outport
  Out2 : Outport  Port=2
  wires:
  Integrator2/1 -> Q eau consommée (ml)/1
  Commutateur/1 -> Débit Humidificateur g/s/1, [Brum_ON]
  In1/1 -> Switch1/1
  Débit Humidificateur g/s/1 -> Mux/2, Mean/1
  Mux/1 -> 1/1
  Mean/1 -> Débit Humidificateur g/s1/1
  Débit Humidificateur g/s1/1 -> Mux/1, Integrator2/1, Out2/1
  Switch1/1 -> Commutateur/1
  [T_int] -> Switch1/2
  Constant/1 -> Switch1/3

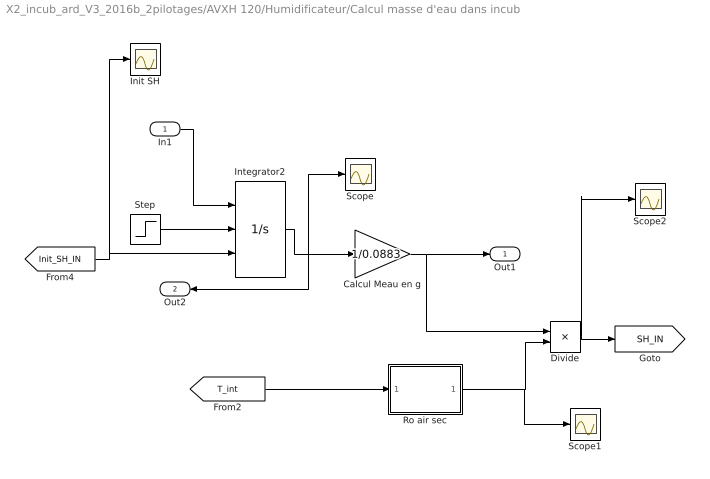
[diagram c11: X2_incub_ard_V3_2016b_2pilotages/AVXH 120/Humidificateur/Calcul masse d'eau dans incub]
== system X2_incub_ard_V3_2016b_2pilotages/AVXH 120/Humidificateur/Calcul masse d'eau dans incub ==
  In1 : Inport
  Calcul Meau en g : Gain  Gain=1/0.0883
  Divide : Product  Inputs=*/
  Init SH : Scope
  Integrator2 : Integrator  ExternalReset=rising  InitialConditionSource=external  InitialCondition=1
  Ro air sec : MATLAB Function  TreatAsAtomicUnit=on
  Scope : Scope
  Scope1 : Scope
  Scope2 : Scope
  Step : Step  SampleTime=0
  Out1 : Outport
  Out2 : Outport  Port=2
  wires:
  Calcul Meau en g/1 -> Divide/1, Out1/1
  In1/1 -> Integrator2/1
  Integrator2/1 -> Scope/1, Calcul Meau en g/1, Out2/1
  Ro air sec/1(ro) -> Scope1/1, Divide/2
  [T_int] -> Ro air sec/1(T)
  Divide/1 -> Scope2/1, [SH_IN]
  [Init_SH_IN] -> Init SH/1, Integrator2/3
  Step/1 -> Integrator2/2

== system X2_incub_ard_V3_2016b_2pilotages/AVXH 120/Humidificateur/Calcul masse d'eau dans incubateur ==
  In1 : Inport
  Calcul Masse eau dans Incub en g : Gain  Gain=0.0883
  Out1 : Outport
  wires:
  In1/1 -> Calcul Masse eau dans Incub en g/1
  Calcul Masse eau dans Incub en g/1 -> Out1/1

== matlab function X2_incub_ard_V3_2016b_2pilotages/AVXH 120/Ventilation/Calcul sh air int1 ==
function [sh,sh2] =CONV_RH_en_SH(T,rh,pl)

% ######################################################################################################
% function [sh]=goff_gratch(T,rh,pl)
%
% fonction de conversion de l'humidité relative ('rh' : en %)
% en humidité spécifique ('sh' : en g/m^3)
% en fonction de :
% la temperature de l'air ('T' : Kelvin, utiliser la fonction C2K si la T est en °C)
% du niveau pression ('pl' : en hPa, si vous avez des matrices 4D, bouclez sur la dimension 
% niveau). 
%
% utilise l'equation de Goff-Gratch pour la determination de
% la tension de vapeur saturante (es) en fonction de la temperature de l'Air
%
% AUTHOR : Nicolas Fauchereau - CRC Dijon - <nicolasf@u-bourgogne.fr>
%
% ######################################################################################################



%Conversion température
T=T+273;


% tension de vapeur saturante
if (T<0), % par rapport a la glace 
eilog = -9.09718 .* ((273.16 ./ T) -1);
eilog2 = -3.5654 .* log10 (273.16 ./ T);
eilog3 = 0.876793 .* (1 - (T ./ 273.16 ));
es=6.1071 .* 10.^(eilog+eilog2+eilog3);

else, % par rapport à l'eau 
eilog=-7.90298 .* ((373.16 ./ T) - 1);
eilog2=5.02808 .* log10((373.16 ./ T));
eilog3=-1.3816e-7 .* ((10.^(11.344.*(1-(T./373.16)))) -1);
eilog4=8.1328e-3 .* ((10.^( -3.49149 .* ((373.16 ./ T) - 1) )) -1);
es=1013.246 .* 10.^(eilog+eilog2+eilog3+eilog4);
end;


% masse
ws = 0.62197 .* es ./ (pl - 0.378.*es);

% masse volumique
ro = 1.293 .* 273 ./ (T);

% humidité spécifique
sh2 = (rh/100.0) .* ws*1000;
sh=sh2*ro; %%% passage en g.m^3

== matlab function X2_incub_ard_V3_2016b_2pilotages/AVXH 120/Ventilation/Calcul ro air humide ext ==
function RO = RO_AIR_HUMIDE(T,P,RH)
P=P*100;
RH=RH/100;
RO = 1/(287.06*(T+273.15))*(P-230.617*RH*exp(17.5043*T/(241.2+T)));

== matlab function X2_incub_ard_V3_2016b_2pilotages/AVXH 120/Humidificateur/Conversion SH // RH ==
function rh  = CONV_SH_en_RH(T,sh,pl)

% ######################################################################################################
% function [sh]=goff_gratch_shtorh(T,sh,pl)
%
% fonction de conversion de l'humidité spécifique ('sh' : en g/m^3)
% en humidité relative ('rh' : %)
% en fonction de :
% la temperature de l'air ('T' : Kelvin, utiliser la fonction C2K si la T est en °C)
% du niveau pression ('pl' : en hPa, si vous avez des matrices 4D, bouclez sur la dimension
% niveau).
%
% utilise l'equation de Goff-Gratch pour la determination de
% la tension de vapeur saturante (es) en fonction de la temperature de l'Air
%
% AUTHOR : Nicolas Fauchereau - CRC Dijon - <nicolasf@u-bourgogne.fr>
%
% ######################################################################################################

%Conversion température
T=T+273;

% tension de vapeur saturante
%if (K2C(T)<0), % par rapport a la glace
if (T<0),
eilog = -9.09718 .* ((273.16 ./ T) -1);
eilog2 = -3.5654 .* log10 (273.16 ./ T);
eilog3 = 0.876793 .* (1 - (T ./ 273.16 ));
es=6.1071 .* 10.^(eilog+eilog2+eilog3);

else, % par rapport à l'eau
eilog=-7.90298 .* ((373.16 ./ T) - 1);
eilog2=5.02808 .* log10((373.16 ./ T));
eilog3=-1.3816e-7 .* ((10.^(11.344.*(1-(T./373.16)))) -1);
eilog4=8.1328e-3 .* ((10.^( -3.49149 .* ((373.16 ./ T) - 1) )) -1);
es=1013.246 .* 10.^(eilog+eilog2+eilog3+eilog4);
end;


% masse
ws = 0.62197 .* es ./ (pl - 0.378.*es);

% masse volumique
ro = 1.293 .* 273 ./ (T);

% humidité relative
rh=(sh./ws) .* 100/(1000*ro);

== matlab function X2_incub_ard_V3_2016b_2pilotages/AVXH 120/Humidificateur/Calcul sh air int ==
function sh =CONV_RH_en_SH(T,rh,pl)

% ######################################################################################################
% function [sh]=goff_gratch(T,rh,pl)
%
% fonction de conversion de l'humidité relative ('rh' : en %)
% en humidité spécifique ('sh' : en g/m^3)
% en fonction de :
% la temperature de l'air ('T' : Kelvin, utiliser la fonction C2K si la T est en °C)
% du niveau pression ('pl' : en hPa, si vous avez des matrices 4D, bouclez sur la dimension 
% niveau). 
%
% utilise l'equation de Goff-Gratch pour la determination de
% la tension de vapeur saturante (es) en fonction de la temperature de l'Air
%
% AUTHOR : Nicolas Fauchereau - CRC Dijon - <nicolasf@u-bourgogne.fr>
%
% ######################################################################################################



%Conversion température
T=T+273.2;


% tension de vapeur saturante
if (T<0), % par rapport a la glace 
eilog = -9.09718 .* ((273.16 ./ T) -1);
eilog2 = -3.5654 .* log10 (273.16 ./ T);
eilog3 = 0.876793 .* (1 - (T ./ 273.16 ));
es=6.1071 .* 10.^(eilog+eilog2+eilog3);

else, % par rapport à l'eau 
eilog=-7.90298 .* ((373.16 ./ T) - 1);
eilog2=5.02808 .* log10((373.16 ./ T));
eilog3=-1.3816e-7 .* ((10.^(11.344.*(1-(T./373.16)))) -1);
eilog4=8.1328e-3 .* ((10.^( -3.49149 .* ((373.16 ./ T) - 1) )) -1);
es=1013.246 .* 10.^(eilog+eilog2+eilog3+eilog4);
end;


% masse
ws = 0.62197 .* es ./ (pl - 0.378.*es);

% masse volumique
ro = 1.293 .* 273 ./ (T);

% humidité spécifique
sh = (rh/100.0)*ws;
sh=sh*1000*ro; %%% passage en g.m^3

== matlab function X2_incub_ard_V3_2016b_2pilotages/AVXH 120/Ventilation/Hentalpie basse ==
function H1 = CALC_HENTALP(T,SH)

H1 =1.006*T+SH*(2500+1.826*T)/1000;

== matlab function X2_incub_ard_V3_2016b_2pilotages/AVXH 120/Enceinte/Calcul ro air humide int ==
function RO = F(T,P,RH)
P=P*100;
RH=RH/100;
RO = 1/(287.06*(T+273.15))*(P-230.617*RH*exp(17.5043*T/(241.2+T)));

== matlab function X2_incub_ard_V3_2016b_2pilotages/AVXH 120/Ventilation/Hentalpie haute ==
function H1 = CALC_HENTALP(T,SH)

H1 =1.006*T+SH*(2500+1.826*T)/1000;

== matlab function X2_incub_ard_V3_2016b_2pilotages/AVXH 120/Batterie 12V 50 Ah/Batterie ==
function [U,E,x] = Batterie(C0, C1, V0, V1, C,I, Icc)
%#codegen


x1=C1/C0;
B=(V1-x1*V0)/(V1*(1-x1));
A=1-B;
x=(C0-C)/C0;
V = V0*(1-(A*(1-x))/(1-B*(1-x)));
U=V-V*I/Icc;
E = U/(1-I/Icc);

== matlab function X2_incub_ard_V3_2016b_2pilotages/AVXH 120/Humidificateur/Calcul masse
d'eau dans incub/Ro air sec ==
function ro = fcn(T)
%#codegen
T=T+273.15;
ro = 1.293 .* 273 ./ (T);

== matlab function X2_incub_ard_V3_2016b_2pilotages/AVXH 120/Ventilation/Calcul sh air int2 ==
function [sh,sh2] =CONV_RH_en_SH(T,rh,pl)

% ######################################################################################################
% function [sh]=goff_gratch(T,rh,pl)
%
% fonction de conversion de l'humidité relative ('rh' : en %)
% en humidité spécifique ('sh' : en g/m^3)
% en fonction de :
% la temperature de l'air ('T' : Kelvin, utiliser la fonction C2K si la T est en °C)
% du niveau pression ('pl' : en hPa, si vous avez des matrices 4D, bouclez sur la dimension 
% niveau). 
%
% utilise l'equation de Goff-Gratch pour la determination de
% la tension de vapeur saturante (es) en fonction de la temperature de l'Air
%
% AUTHOR : Nicolas Fauchereau - CRC Dijon - <nicolasf@u-bourgogne.fr>
%
% ######################################################################################################



%Conversion température
T=T+273;


% tension de vapeur saturante
if (T<0), % par rapport a la glace 
eilog = -9.09718 .* ((273.16 ./ T) -1);
eilog2 = -3.5654 .* log10 (273.16 ./ T);
eilog3 = 0.876793 .* (1 - (T ./ 273.16 ));
es=6.1071 .* 10.^(eilog+eilog2+eilog3);

else, % par rapport à l'eau 
eilog=-7.90298 .* ((373.16 ./ T) - 1);
eilog2=5.02808 .* log10((373.16 ./ T));
eilog3=-1.3816e-7 .* ((10.^(11.344.*(1-(T./373.16)))) -1);
eilog4=8.1328e-3 .* ((10.^( -3.49149 .* ((373.16 ./ T) - 1) )) -1);
es=1013.246 .* 10.^(eilog+eilog2+eilog3+eilog4);
end;


% masse
ws = 0.62197 .* es ./ (pl - 0.378.*es);

% masse volumique
ro = 1.293 .* 273 ./ (T);

% humidité spécifique
sh2 = (rh/100.0) .* ws*1000;
sh=sh2*ro; %%% passage en g.m^3

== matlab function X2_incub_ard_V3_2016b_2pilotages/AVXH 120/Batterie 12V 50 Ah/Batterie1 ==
function [U,E,x] = Batterie(C0, C1, V0, V1, C,I, Icc)
%#codegen


x1=C1/C0;
B=(V1-x1*V0)/(V1*(1-x1));
A=1-B;
x=(C0-C)/C0;
V = V0*(1-(A*(1-x))/(1-B*(1-x)));
U=V-V*I/Icc;
E = U/(1-I/Icc);
